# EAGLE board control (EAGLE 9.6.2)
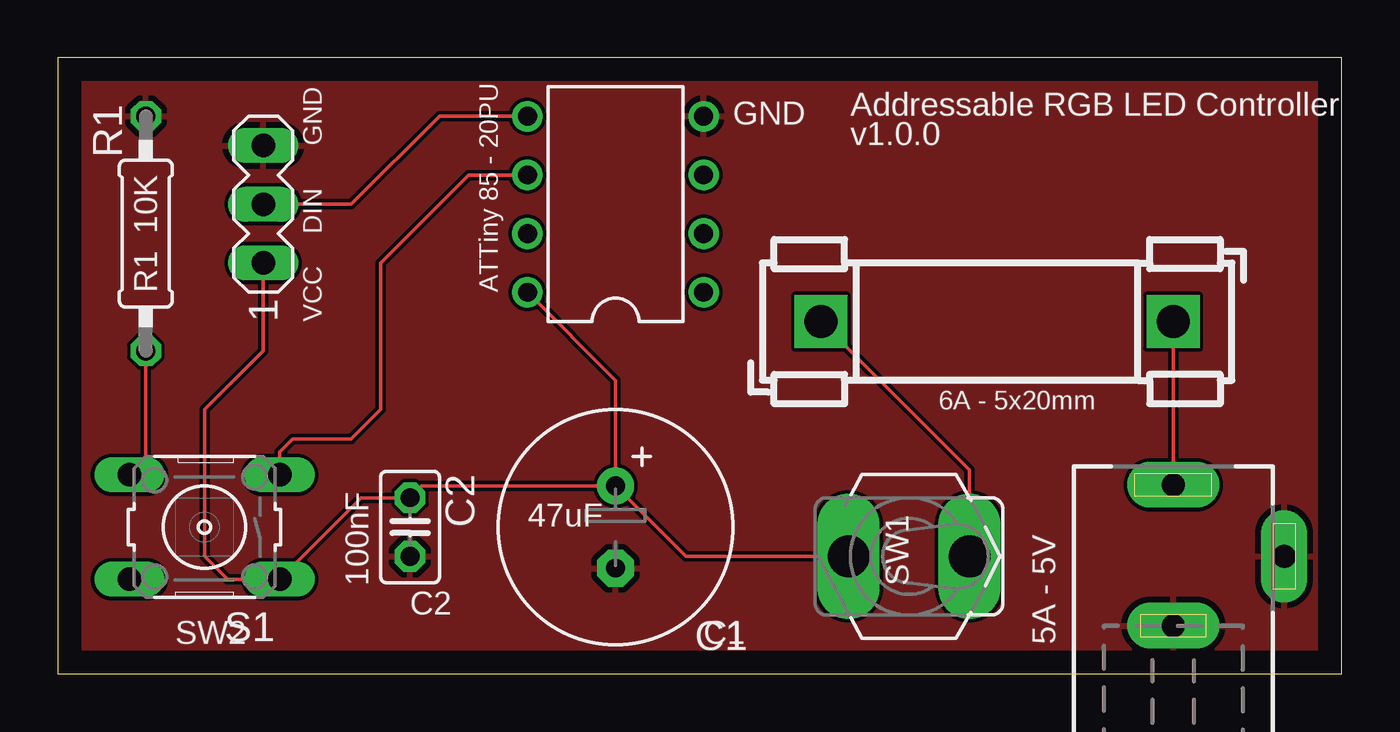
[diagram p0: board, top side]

Size 55.55 x 26.66 mm. Coordinates in mm from the lower left corner, seen from the top.
Outline: 0,0 55.55,0 55.55,26.66 0,26.66 0,0
Copper layers (1*16): Top 0.035mm / dielectric 1.5mm / Bottom 0.035mm
Design rules "default": minimum track width 6mil, minimum drill 0.35mm, track to track 6mil, track to pad 6mil, pad to pad 6mil, via to via 6mil, smd to smd 6mil, copper to edge 40mil, drill to drill 6mil, minimum pad ring 10mil, minimum via ring 8mil, stop-mask expansion 4mil, vias tented up to drill 0mil, thermal gap 10mil

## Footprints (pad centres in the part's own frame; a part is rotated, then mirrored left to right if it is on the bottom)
PDIP08_300MIL = drill 0.813: 1 -3.81,-3.81; 2 -1.27,-3.81; 3 1.27,-3.81; 4 3.81,-3.81; 5 3.81,3.81; 6 1.27,3.81; 7 -1.27,3.81; 8 -3.81,3.81
E3,5-10 = drill 0.813 pad 1.6: + -1.778,0 | drill 0.813 pad 1.6 octagon: - 1.778,0
C025-025X050 = drill 0.813 octagon: 1 -1.27,0; 2 1.27,0
DCJ0303 = drill 1 pad 2 long: 1 0,3.1; 2 4.8,0; 3 0,-3
FUSE_HOLDER_5X20MM = drill 1.422 pad 2.286 square: 1 0,0; 2 15.24,0
MA03-1 = drill 1.016 long: 1 -2.54,0; 2 0,0; 3 2.54,0
0207/10 = drill 0.813 octagon: 1 -5.08,0; 2 5.08,0
B3F-10XX = drill 1.016 long: 1 -3.251,2.261; 2 3.251,2.261; 3 -3.251,-2.261; 4 3.251,-2.261
MS243 = drill 1.803 pad 2 long: 1 0,-3.886; 2 0,1.346

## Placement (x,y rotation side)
ATTINY_85  ATTINY85-20P  [PDIP08_300MIL]  24.13,20.32 90 top
C1  47uF  [E3,5-10]  24.13,6.35 270 top
C2  100nF  [C025-025X050]  15.24,6.35 270 top
DC-2.1X5.5MM  5V 5A  [DCJ0303]  48.26,5.08 0 top
FUSE_6A_5X20  FUSEBLANK_5X20MM  [FUSE_HOLDER_5X20MM]  48.26,15.24 180 top
LEDSTRIP  [MA03-1]  8.89,20.32 90 top
R1  10K  [0207/10]  3.81,19.05 270 top
S1  [B3F-10XX]  6.35,6.35 180 top
SWITCH  [MS243]  35.56,5.08 90 top

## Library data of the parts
ATTINY_85 = _hhn_attiny25_45_85
C1 C2 = rcl; SPICEPREFIX: C
DC-2.1X5.5MM = con-jack; OC_FARNELL: unknown; OC_NEWARK: unknown
FUSE_6A_5X20 = fuse; OC_FARNELL: unknown; OC_NEWARK: unknown
LEDSTRIP = con-lstb; OC_FARNELL: unknown; OC_NEWARK: unknown
R1 = rcl; SPICEPREFIX: R
S1 = switch-omron; MPN: B3F-1000; OC_FARNELL: 176432; OC_NEWARK: 36M3542
SWITCH = fixed-switch

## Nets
DATAIN: ATTINY_85.5 LEDSTRIP.2
GND: ATTINY_85.4 C1.- C2.2 DC-2.1X5.5MM.2 DC-2.1X5.5MM.3 LEDSTRIP.3 R1.1
N$3: R1.2 S1.4
N$4: DC-2.1X5.5MM.1 FUSE_6A_5X20.1
N$5: FUSE_6A_5X20.2 SWITCH.1
SWITCHIN: ATTINY_85.6 S1.3
VCC: ATTINY_85.8 C1.+ C2.1 LEDSTRIP.1 S1.1 SWITCH.2

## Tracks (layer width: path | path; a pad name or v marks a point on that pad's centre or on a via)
DATAIN
  Top 0.152: LEDSTRIP.2 12.7,20.32 16.51,24.13 ATTINY_85.5
GND
  pour Top: 0,0 0,26.67 55.88,26.67 55.88,0
N$3
  Top 0.152: R1.2 3.81,9.32 S1.4
N$4
  Top 0.152: DC-2.1X5.5MM.1 FUSE_6A_5X20.1
N$5
  Top 0.152: FUSE_6A_5X20.2 39.45,8.81 SWITCH.1
SWITCHIN
  Top 0.152: ATTINY_85.6 17.78,21.59 13.97,17.78 13.97,11.43 12.7,10.16 10.16,10.16 9.6,9.6 S1.3
VCC
  Top 0.152: LEDSTRIP.1 8.89,13.97 6.35,11.43 6.35,5.08 7.34,4.09 S1.1 13.13,7.62 C2.1 15.75,8.13 C1.+ | ATTINY_85.8 24.13,12.7 C1.+ | C1.+ 27.18,5.08 SWITCH.2

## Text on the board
tPlace: GND | Addressable RGB LED Controller | GND | v1.0.0 | 10K | DIN | R1 | ATTiny 85 - 20PU | VCC | 6A - 5x20mm | 47uF | 100nF | SW1 | C2 | SW2 | C1 | 5A - 5V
